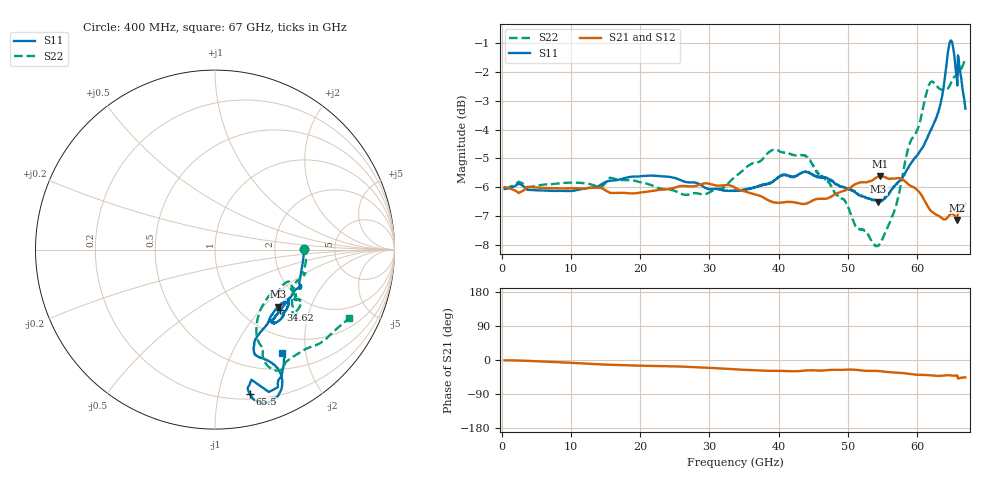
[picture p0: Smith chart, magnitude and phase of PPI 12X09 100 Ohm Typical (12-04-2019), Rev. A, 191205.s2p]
!Keysight Technologies,N5227A,US56070614,A.10.47.06
!Date:	12/4/2019
!Correction
!S11(Full 2 Port(1,2))
!S21(Full 2 Port(1,2))
!S12(Full 2 Port(1,2))
!S22(Full 2 Port(1,2))
!S2P File: Measurements: S11, S21, S12, S22
# GHz S  dB  R 50
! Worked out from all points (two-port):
!   801 points, 400 MHz to 67 GHz, reference 50 ohm
!   highest |S21| = -5.61 dB at 54.68 GHz (marker M1); lowest = -7.1 dB at 65.83 GHz (marker M2)
!   |S21| within 3 dB of the highest: start of sweep to end of sweep
!   lowest |S11| = -6.5 dB at 54.43 GHz (marker M3), VSWR 2.80, Z = 74.3 - j60.8 ohm
!   |S11| at or under -10 dB: nowhere
!   |S22| runs from -8.0 to -1.5 dB; largest |S21 - S12| = 0.005
!   S11 on the Smith chart (normalised r, x): 400 MHz: 2.98, +0.02; 34.62 GHz: 1.46, -1.30; 65.5 GHz: 0.25, -1.24; 67 GHz: 0.74, -1.60
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0.4  -6.06 0.4  -5.99 -0.8  -5.98 -0.7  -6.05 0.4
11.56  -6.07 -15.9  -6.04 -9.1  -6.02 -9.1  -5.85 -10.0
17.8  -5.68 -24.7  -6.20 -14.1  -6.17 -14.2  -5.75 -17.4
22.63  -5.61 -23.6  -6.09 -16.0  -6.07 -16.1  -6.02 -19.4
28.79  -5.93 -25.6  -5.89 -19.3  -5.86 -19.4  -6.24 -24.4
33.7  -6.13 -39.9  -6.01 -24.6  -5.97 -24.7  -5.64 -34.8
34.62  -6.09 -42.7  -6.11 -25.4  -6.08 -25.6  -5.46 -35.9
38.78  -5.88 -51.7  -6.48 -28.5  -6.45 -28.6  -4.76 -39.0
44.86  -5.57 -43.8  -6.47 -27.1  -6.43 -27.2  -5.21 -30.7
50.52  -6.12 -34.0  -6.00 -25.1  -5.95 -25.3  -7.01 -23.4
54.43  -6.50 -42.1  -5.63 -29.0  -5.59 -29.3  -8.03 -42.7
54.68  -6.47 -43.4  -5.61 -29.5  -5.56 -29.8  -7.94 -45.3
55.93  -6.21 -51.0  -5.71 -32.1  -5.65 -32.3  -7.30 -55.4
60.51  -4.73 -68.1  -6.22 -39.2  -6.18 -39.7  -3.66 -66.0
61.67  -4.19 -69.2  -6.71 -40.0  -6.67 -40.4  -2.49 -63.6
63.42  -3.10 -63.8  -7.04 -41.7  -7.01 -42.1  -2.60 -57.8
64.25  -1.76 -62.6  -7.09 -40.3  -7.06 -40.7  -2.61 -52.3
64.92  -0.91 -70.5  -6.93 -40.8  -6.90 -41.1  -2.38 -45.4
65.5  -1.67 -76.5  -7.01 -41.5  -6.98 -41.8  -2.14 -42.4
65.83  -2.47 -74.4  -7.13 -40.6  -7.10 -40.9  -2.09 -41.1
66.33  -2.10 -61.6  -6.84 -46.9  -6.80 -47.2  -1.93 -35.5
67  -3.27 -56.8  -6.58 -46.0  -6.55 -46.4  -1.52 -27.1
